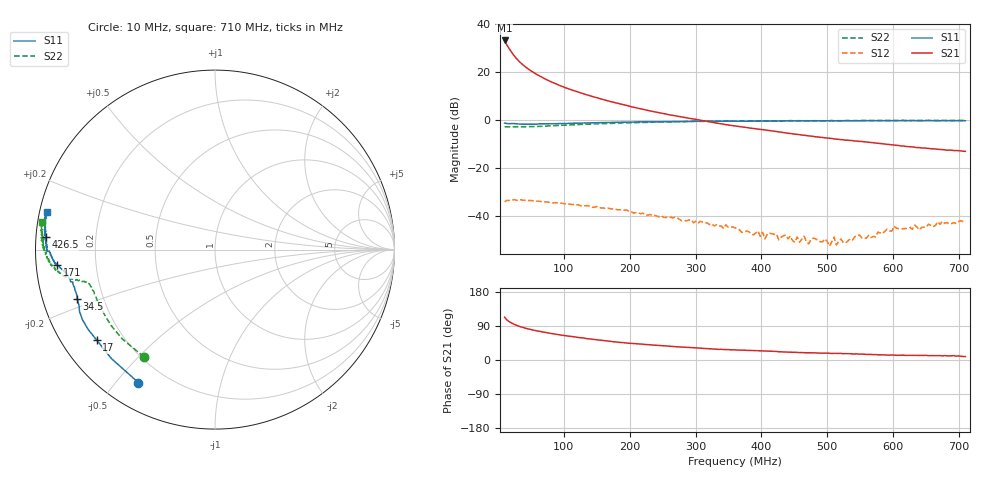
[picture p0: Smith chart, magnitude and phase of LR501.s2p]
!  POLYFET RF DEVICES
!  LR501 (Each Side)
!  S PARAMETERS
!  VDS=28V, IDQ=400mA
! Date: Thu Mar 13 09:54:24 2003
# MHZ S MA R 50
! Freq=Mhz Mag[s11] Ang[s11] Mag[s21] Ang[s21] Mag[s12] Ang[s12] Mag[s22] Ang[s22]
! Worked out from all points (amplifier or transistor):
!   201 points, 10 MHz to 710 MHz, reference 50 ohm
!   highest |S21| = 33.2 dB at 10 MHz (marker M1)
!   |S21| within 3 dB of that: start of sweep to 15.97 MHz
!   unconditionally stable (mu >= 1): 368.1 MHz to 408.6 MHz; 411.7 MHz to 443.8 MHz; 444.1 MHz to end of sweep
!   at 125.5 MHz: K = 0.20, MSG = 23.6 dB, |S12| = -35.9 dB
!   at 360 MHz: K = 0.82, MSG = 21.3 dB, |S12| = -45.1 dB
!   at 710 MHz: K = 1.47, MAG = 10.7 dB, |S12| = -42.8 dB
!   S11 on the Smith chart (normalised r, x): 10 MHz: 0.10, -0.57; 17 MHz: 0.10, -0.34; 34.5 MHz: 0.10, -0.17; 171 MHz: 0.06, -0.05; 426.5 MHz: 0.03, +0.04; 710 MHz: 0.02, +0.11
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10  0.8552 -119.9  45.46 112.8  0.01944 23.6  0.717 -123.5
13.5  0.8376 -133.6  36.45 105.6  0.02076 15.3  0.7173 -136.2
17  0.8297 -142.6  30.56 101.1  0.02073 8.9  0.7171 -144.0
20.5  0.8353 -148.1  25.87 97.7  0.02089 9.0  0.7146 -149.2
24  0.8353 -152.1  22.3 94.6  0.02157 4.6  0.7133 -153.2
27.5  0.8298 -155.5  19.47 91.9  0.02098 0.4  0.7157 -156.0
31  0.8186 -157.8  17.27 89.4  0.02067 -1.6  0.7136 -158.0
34.5  0.8155 -160.3  15.46 87.6  0.02143 -3.5  0.7162 -159.8
41.5  0.8104 -163.2  12.8 84.0  0.02089 -5.2  0.7185 -161.7
48.5  0.8109 -164.8  10.86 81.1  0.02069 -7.4  0.7228 -163.5
59  0.813 -167.2  8.829 76.9  0.02002 -10.8  0.7259 -164.8
69.5  0.8222 -168.3  7.393 73.4  0.0195 -14.4  0.7346 -165.5
94  0.8339 -170.6  5.187 66.2  0.01851 -21.3  0.7643 -166.9
129  0.86 -172.6  3.532 58.2  0.01585 -25.6  0.8054 -167.9
171  0.8843 -174.3  2.404 49.2  0.01399 -32.2  0.8437 -169.7
244.5  0.9094 -177.5  1.41 38.2  0.00946 -34.8  0.8965 -173.0
360  0.9394 178.2  0.743 26.7  0.00555 -31.8  0.9385 -178.2
426.5  0.9466 175.8  0.5584 21.8  0.00312 -3.3  0.953 179.6
479  0.954 174.1  0.4514 18.8  0.0034 8.1  0.9587 177.5
503.5  0.9583 173.4  0.4138 17.7  0.0023 25.3  0.9562 177.0
594.5  0.9582 170.5  0.3039 12.9  0.00482 63.1  0.9713 174.3
710  0.9584 167.5  0.2195 9.2  0.00728 80.6  0.9776 171.1
